FUNCTION "Gest Auto 2ndCC" : VOID
TITLE =GESTIONE AUTOMATICO 2nd CONTROLLO CORTI
VERSION : 0.1

BEGIN
NETWORK
TITLE =Start ciclo automatico
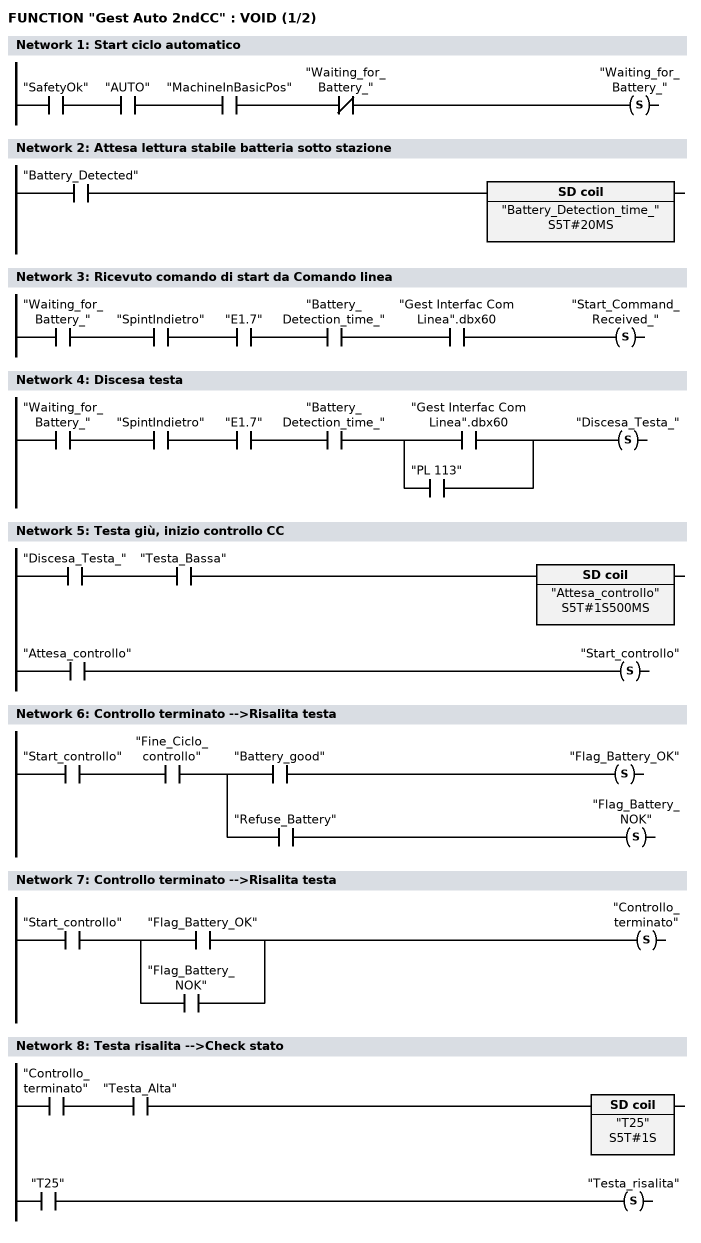
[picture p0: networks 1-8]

      U     "SafetyOk";
      U     "AUTO";
      U     "MachineInBasicPos";
      UN    "Waiting_for_Battery_";
      S     "Waiting_for_Battery_";
NETWORK
TITLE =Attesa lettura stabile batteria sotto stazione

      U     "Battery_Detected";
      L     S5T#20MS;
      SE    "Battery_Detection_time_";
      NOP   0;
      NOP   0;
      NOP   0;
      NOP   0;
NETWORK
TITLE =Ricevuto comando di start da Comando linea

      U     "Waiting_for_Battery_";
      U     "SpintIndietro";
      U     "E1.7";
      U     "Battery_Detection_time_";
      U     "Gest Interfac Com Linea".dbx60;
      S     "Start_Command_Received_";
NETWORK
TITLE =Discesa testa

      U     "Waiting_for_Battery_";
      U     "SpintIndietro";
      U     "E1.7";
      U     "Battery_Detection_time_";
      U(    ;
      O     "Gest Interfac Com Linea".dbx60;
      O     "PL 113";
      )     ;
      S     "Discesa_Testa_";
NETWORK
TITLE =Testa giù, inizio controllo CC

      U     "Discesa_Testa_";
      U     "Testa_Bassa";
      L     S5T#1S500MS;
      SE    "Attesa_controllo";
      NOP   0;
      NOP   0;
      NOP   0;
      U     "Attesa_controllo";
      S     "Start_controllo";
NETWORK
TITLE =Controllo terminato -->Risalita testa

      U     "Start_controllo";
      U     "Fine_Ciclo_controllo";
      =     L      0.0;
      U     L      0.0;
      U     "Battery_good";
      S     "Flag_Battery_OK";
      U     L      0.0;
      U     "Refuse_Battery";
      S     "Flag_Battery_NOK";
NETWORK
TITLE =Controllo terminato -->Risalita testa

      U     "Start_controllo";
      U(    ;
      O     "Flag_Battery_OK";
      O     "Flag_Battery_NOK";
      )     ;
      S     "Controllo_terminato";
NETWORK
TITLE =Testa risalita -->Check stato

      U     "Controllo_terminato";
      U     "Testa_Alta";
      L     S5T#1S;
      SE    "T25";
      NOP   0;
      NOP   0;
      NOP   0;
      U     "T25";
      S     "Testa_risalita";
NETWORK
TITLE =Se la batteria non è buona viene attivato lo scarto
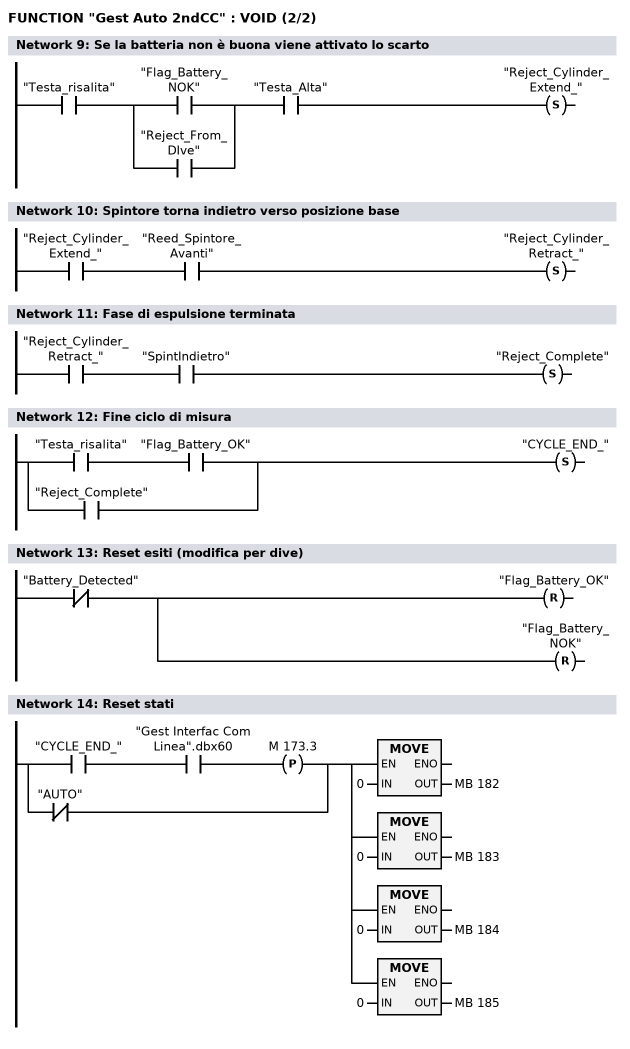
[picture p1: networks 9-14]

      U     "Testa_risalita";
      U(    ;
      O     "Flag_Battery_NOK";
      O     "Reject_From_DIve";
      )     ;
      U     "Testa_Alta";
      S     "Reject_Cylinder_Extend_";
NETWORK
TITLE =Spintore torna indietro verso posizione base

      U     "Reject_Cylinder_Extend_";
      U     "Reed_Spintore_Avanti";
      S     "Reject_Cylinder_Retract_";
NETWORK
TITLE =Fase di espulsione terminata

      U     "Reject_Cylinder_Retract_";
      U     "SpintIndietro";
      S     "Reject_Complete";
NETWORK
TITLE =Fine ciclo di misura

      U     "Testa_risalita";
      U     "Flag_Battery_OK";
      O     "Reject_Complete";
      S     "CYCLE_END_";
NETWORK
TITLE =Reset esiti (modifica per dive)

      UN    "Battery_Detected";
      R     "Flag_Battery_OK";
      R     "Flag_Battery_NOK";
NETWORK
TITLE =Reset stati

      U     "CYCLE_END_";
      U     "Gest Interfac Com Linea".dbx60;
      FP    M    173.3;
      ON    "AUTO";
      =     L      0.0;
      U     L      0.0;
      SPBNB _001;
      L     0;
      T     MB   182;
_001: NOP   0;
      U     L      0.0;
      SPBNB _002;
      L     0;
      T     MB   183;
_002: NOP   0;
      U     L      0.0;
      SPBNB _003;
      L     0;
      T     MB   184;
_003: NOP   0;
      U     L      0.0;
      SPBNB _004;
      L     0;
      T     MB   185;
_004: NOP   0;
END_FUNCTION

